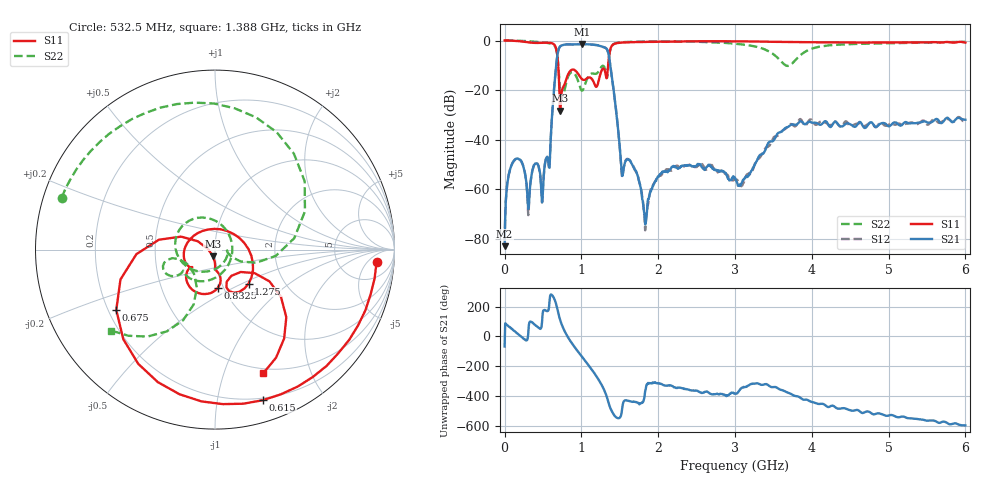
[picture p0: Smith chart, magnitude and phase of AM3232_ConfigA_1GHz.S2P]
! Network Analyzer HP8753E.07.74: Oct 30, 2002 Serial No. US37390186
! 13 Jul 2023  12:30:17
! Frequency  S11  S21  S12  S22
# HZ  S  DB R  50
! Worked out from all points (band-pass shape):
!   801 points, 30 kHz to 6 GHz, reference 50 ohm
!   highest |S21| = -1.39 dB at 1.005 GHz (marker M1); lowest = -83.1 dB at 30 kHz (marker M2)
!   |S21| within 3 dB of the highest: 696.6 MHz to 1.344 GHz (647 MHz wide, 63.4 % of centre)
!   lowest |S11| = -28.3 dB at 727.5 MHz (marker M3), VSWR 1.08, Z = 48.7 - j3.54 ohm
!   |S11| at or under -10 dB: 697.6 MHz to 1.348 GHz (649.9 MHz wide, 63.6 % of centre)
!   |S22| runs from -23.6 to 0.0 dB; largest |S21 - S12| = 0.016
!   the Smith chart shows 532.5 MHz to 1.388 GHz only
!   S11 on the Smith chart (normalised r, x): 532.5 MHz: 13, -9; 615 MHz: 0.18, -1.35; 675 MHz: 0.23, -0.27; 832.5 MHz: 0.94, -0.42; 1.275 GHz: 1.33, -0.54; 1.388 GHz: 0.45, -1.37
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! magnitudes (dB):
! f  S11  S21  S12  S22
! 30 kHz  0.0  -83.1  -80.8  0.0
! 52.53 MHz  0.0  -54.3  -54.4  0.0
! 120 MHz  -0.1  -48.6  -48.7  0.0
! 307.5 MHz  -0.7  -68.1  -70.5  -0.3
! 390 MHz  -1.0  -50.1  -50.0  -0.5
! 532.5 MHz  -0.9  -48.7  -48.5  -0.9
! 615 MHz  -1.1  -31.7  -31.5  -1.4
! 675 MHz  -3.8  -9.0  -8.9  -4.0
! 727.5 MHz  -28.3  -2.3  -2.3  -22.6
! 832.5 MHz  -13.3  -1.6  -1.6  -14.2
! 1.005 GHz  -15.5  -1.4  -1.4  -20.3
! 1.275 GHz  -11.5  -2.5  -2.6  -10.2
! 1.388 GHz  -2.6  -12.6  -12.8  -2.7
! 1.538 GHz  -0.8  -54.5  -54.4  -0.7
! 1.688 GHz  -0.7  -51.6  -51.5  -0.5
! 1.838 GHz  -0.6  -73.8  -74.3  -0.4
! 2.003 GHz  -0.5  -55.2  -54.5  -0.4
! 3 GHz  -0.3  -55.4  -56.1  -1.3
! 3.683 GHz  -0.6  -35.0  -34.8  -10.3
! 4.005 GHz  -0.7  -33.2  -32.4  -3.2
! 5.003 GHz  -0.8  -34.7  -34.0  -1.1
! 6 GHz  -0.9  -32.0  -32.2  -0.5
